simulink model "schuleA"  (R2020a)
settings: Solver=FixedStepDiscrete  StartTime=0.0  StopTime=8  FixedStep=1  RelTol=1e-3  EnableMultiTasking=on

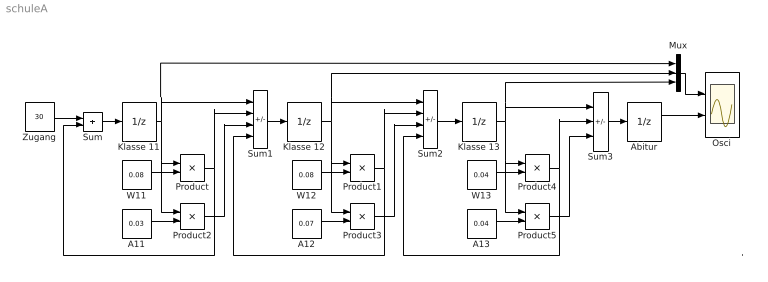
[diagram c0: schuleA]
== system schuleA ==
  note: .
  A11 : Constant  Value=0.03
  A12 : Constant  Value=0.07
  A13 : Constant  Value=0.04
  Abitur : UnitDelay  SampleTime=-1  HasFrameUpgradeWarning=on
  Klasse 11 : UnitDelay  SampleTime=-1  HasFrameUpgradeWarning=on
  Klasse 12 : UnitDelay  SampleTime=-1  HasFrameUpgradeWarning=on
  Klasse 13 : UnitDelay  SampleTime=-1  HasFrameUpgradeWarning=on
  Mux : Mux  Inputs=3
  Osci : Scope  NumInputPorts=2
  Product{,1..5} (6 alike) : Product  InputSameDT=on  RndMeth=Zero  SaturateOnIntegerOverflow=on
  Sum : Sum  InputSameDT=on  SaturateOnIntegerOverflow=on
  Sum1 : Sum  Inputs=+--+  InputSameDT=on  SaturateOnIntegerOverflow=on
  Sum2 : Sum  Inputs=+--+  InputSameDT=on  SaturateOnIntegerOverflow=on
  Sum3 : Sum  Inputs=+--  InputSameDT=on  SaturateOnIntegerOverflow=on
  W11 : Constant  Value=0.08
  W12 : Constant  Value=0.08
  W13 : Constant  Value=0.04
  Zugang : Constant  Value=30
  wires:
  Zugang/1 -> Sum/1
  Sum/1 -> Klasse 11/1
  Sum1/1 -> Klasse 12/1
  W11/1 -> Product/2
  Klasse 11/1 -> Product/1, Product2/1, Sum1/1, Mux/1
  A11/1 -> Product2/2
  Product/1 -> Sum/2, Sum1/2
  Product2/1 -> Sum1/3
  W12/1 -> Product1/2
  Klasse 12/1 -> Product1/1, Product3/1, Sum2/1, Mux/2
  A12/1 -> Product3/2
  Sum2/1 -> Klasse 13/1
  W13/1 -> Product4/2
  Klasse 13/1 -> Product4/1, Product5/1, Sum3/1, Mux/3
  A13/1 -> Product5/2
  Product1/1 -> Sum2/2, Sum1/4
  Product3/1 -> Sum2/3
  Product4/1 -> Sum2/4, Sum3/2
  Product5/1 -> Sum3/3
  Mux/1 -> Osci/1
  Sum3/1 -> Abitur/1
  Abitur/1 -> Osci/2
